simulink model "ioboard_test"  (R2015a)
settings: Solver=FixedStepDiscrete  StartTime=0.0  StopTime=40  FixedStep=0.0001  RelTol=1e-3
libraries: slrtlib x3, xpcnilib x2

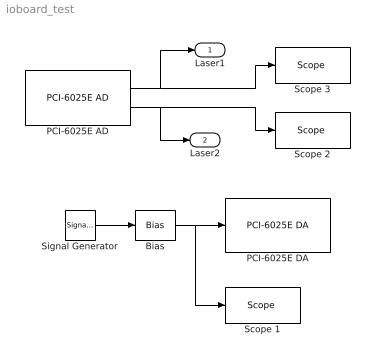
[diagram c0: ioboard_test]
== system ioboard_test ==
  Bias : Bias  Bias=1.5
  PCI-6025E AD : xpcnilib/A//D/E Series/PCI-6025E AD  channel=[1 2]  range=[-5 -5]  coupling=[0 0]  sampletime=0.0001  slot=-1
  PCI-6025E DA : xpcnilib/D//A/E Series/PCI-6025E DA  channel=[1]  reset=[1]  initValue=[0]  sampletime=0.0001  slot=-1
  Scope 1 : slrtlib/Displays and Logging/Scope   scopeno=3  scopetype=Target  autostart=on  viewmode=Graphical sliding  formatstr='%15.6f'  grid=on  ylimits=[-1 8]  nosamples=1000  noprepostsamples=0  interleave=100  triggermode=FreeRun  triggersignal=1  trigsignalfromport=off  triggerlevel=0.0  triggerslope=Either  triggerscope=1  triggersample=0  filename=data.dat  mode=Lazy  writesize=512  autorestart=off  dynamicfilemode=off  maxwritefilesize=512*1024^2
  Scope 2 : slrtlib/Displays and Logging/Scope   scopeno=1  scopetype=Target  autostart=on  viewmode=Graphical sliding  formatstr='%15.6f'  grid=on  ylimits=[-1,6]  nosamples=1000  noprepostsamples=0  interleave=100  triggermode=FreeRun  triggersignal=1  trigsignalfromport=off  triggerlevel=0.0  triggerslope=Either  triggerscope=1  triggersample=0  filename=data.dat  mode=Lazy  writesize=512  autorestart=off  dynamicfilemode=off  maxwritefilesize=512*1024^2
  Scope 3 : slrtlib/Displays and Logging/Scope   scopeno=4  scopetype=Target  autostart=on  viewmode=Graphical sliding  formatstr='%15.6f'  grid=on  ylimits=[-1,6]  nosamples=1000  noprepostsamples=0  interleave=100  triggermode=FreeRun  triggersignal=1  trigsignalfromport=off  triggerlevel=0.0  triggerslope=Either  triggerscope=1  triggersample=0  filename=data.dat  mode=Lazy  writesize=512  autorestart=off  dynamicfilemode=off  maxwritefilesize=512*1024^2
  Signal Generator : SignalGenerator  WaveForm=sawtooth  Amplitude=1.5  Frequency=0.2
  Laser1 : Outport
  Laser2 : Outport  Port=2
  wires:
  Signal Generator/1 -> Bias/1
  Bias/1 -> Scope 1/1, PCI-6025E DA/1
  PCI-6025E AD/1 -> Laser1/1, Scope 3/1
  PCI-6025E AD/2 -> Laser2/1, Scope 2/1
